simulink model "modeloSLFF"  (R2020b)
settings: Solver=VariableStepAuto  StartTime=0.0  StopTime=160.0  RelTol=1e-3
PreLoadFcn:
  | s=tf('s');
  | G_t2t1_sinret=(0.55/(0.25*s+1)^2+0.35/(2.7*s+1)^2);
  | G_t2t1=exp(-1.5*s)*G_t2t1_sinret;
  | G_t2u_sinret=1.1/(2.6*s+1)^3;
  | G_t2u=exp(-.45*s)*G_t2u_sinret;
libraries: simulink x3, cstblocks x2

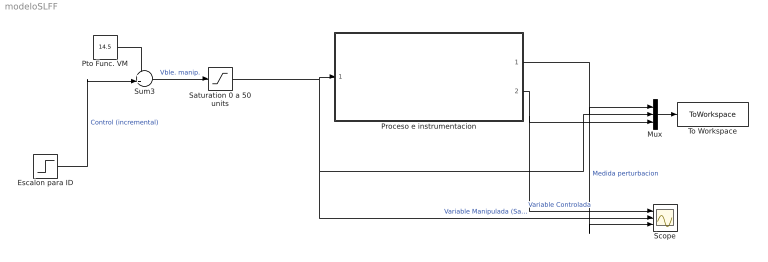
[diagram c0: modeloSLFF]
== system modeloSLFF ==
  Escalon para ID : Step  Time=40  After=15  SampleTime=0
  Mux : Mux  Inputs=3
  Proceso e instrumentacion : Subsystem
  Pto Func. VM : Constant  Value=14.5
  Saturation 0 a 50 units : Saturate  UpperLimit=50  LowerLimit=0
  Scope : Scope  NumInputPorts=3
  Sum3 : Sum  Inputs=++|
  To Workspace : ToWorkspace  VariableName=simout  SampleTime=-1
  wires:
  Proceso e instrumentacion/2(Out2) -> Scope/1, Mux/3  "Variable Controlada"
  Sum3/1 -> Saturation 0 a 50 units/1  "Vble. manip."
  Proceso e instrumentacion/1(Out1) -> Scope/3, Mux/1  "Medida perturbacion"
  Pto Func. VM/1 -> Sum3/1
  Escalon para ID/1 -> Sum3/2  "Control (incremental)"
  Mux/1 -> To Workspace/1
  Saturation 0 a 50 units/1 -> Scope/2, Mux/2, Proceso e instrumentacion/1(In2)  "Variable Manipulada (Sat.)"

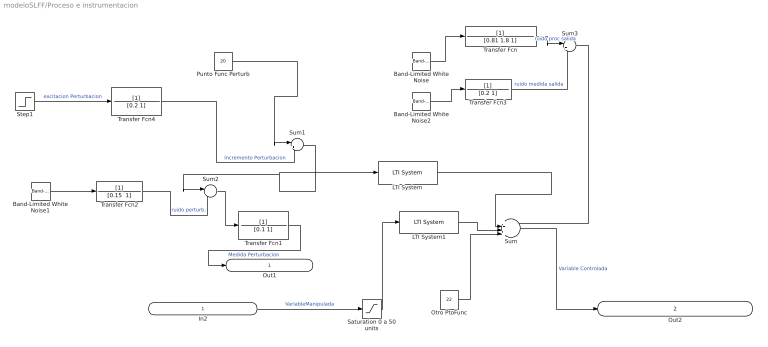
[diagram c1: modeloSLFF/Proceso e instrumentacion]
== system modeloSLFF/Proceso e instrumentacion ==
  In2 : Inport
  Band-Limited White Noise : simulink/Sources/Band-Limited White Noise  Cov=[4.5]  Ts=0.3  seed=[231]
  Band-Limited White Noise1 : simulink/Sources/Band-Limited White Noise  Cov=[0.015]  Ts=0.1  seed=[341]
  Band-Limited White Noise2 : simulink/Sources/Band-Limited White Noise  Cov=[0.025]  Ts=0.1  seed=[23341]
  LTI System : cstblocks/LTI System  sys=G_t2t1  IC=[]
  LTI System1 : cstblocks/LTI System  sys=G_t2u  IC=[]
  Otro PtoFunc : Constant  Value=22
  Punto Func Perturb : Constant  Value=20
  Saturation 0 a 50 units : Saturate  UpperLimit=50  LowerLimit=0
  Step1 : Step  Time=100  After=15  SampleTime=0
  Sum : Sum  Inputs=++++|
  Sum1 : Sum  Inputs=|++
  Sum2 : Sum  Inputs=|++
  Sum3 : Sum  Inputs=|++
  Transfer Fcn : TransferFcn  Denominator=[0.81 1.8 1]
  Transfer Fcn1 : TransferFcn  Denominator=[0.1 1]
  Transfer Fcn2 : TransferFcn  Denominator="[0.15  1]"
  Transfer Fcn3 : TransferFcn  Denominator=[0.2 1]
  Transfer Fcn4 : TransferFcn  Denominator=[0.2 1]
  Out1 : Outport
  Out2 : Outport  Port=2
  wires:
  LTI System1/1 -> Sum/3
  Band-Limited White Noise/1 -> Transfer Fcn/1
  Transfer Fcn2/1 -> Sum2/2  "ruido perturb."
  Band-Limited White Noise1/1 -> Transfer Fcn2/1
  Punto Func Perturb/1 -> Sum1/1
  Sum/1 -> Out2/1  "Variable Controlada"
  Sum1/1 -> LTI System/1, Sum2/1
  LTI System/1 -> Sum/2
  Saturation 0 a 50 units/1 -> LTI System1/1
  In2/1 -> Saturation 0 a 50 units/1  "VariableManipulada"
  Otro PtoFunc/1 -> Sum/4
  Transfer Fcn1/1 -> Out1/1  "Medida Perturbacion"
  Sum2/1 -> Transfer Fcn1/1
  Transfer Fcn/1 -> Sum3/1  "ruido proc salida"
  Transfer Fcn3/1 -> Sum3/2  "ruido medida salida"
  Sum3/1 -> Sum/1
  Band-Limited White Noise2/1 -> Transfer Fcn3/1
  Step1/1 -> Transfer Fcn4/1  "excitacion Perturbacion"
  Transfer Fcn4/1 -> Sum1/2  "Incremento Perturbacion"
